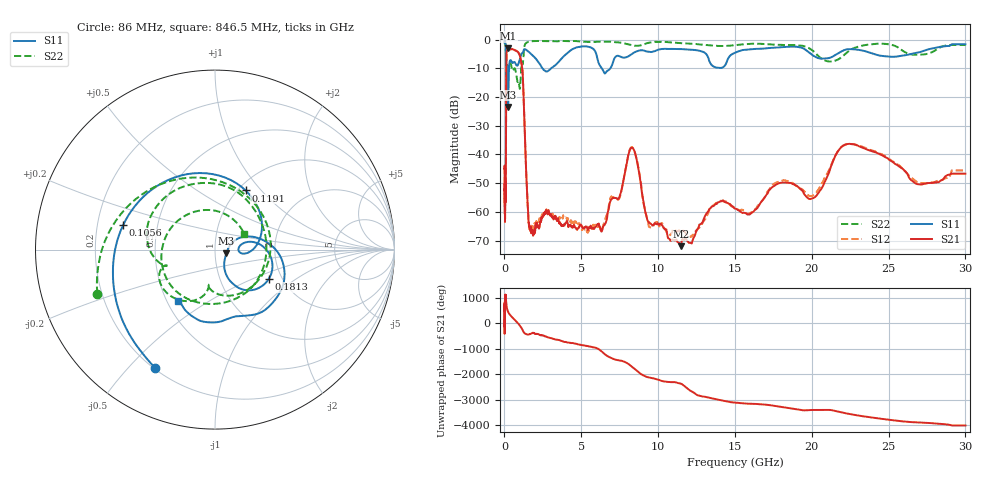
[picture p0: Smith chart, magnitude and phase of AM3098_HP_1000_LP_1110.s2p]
! Date/Time: Thu, Feb 28, 2019 8:40 AM
! Network Analyzer: Agilent Technologies E8364B Rev: A.07.50.67
! Sweep from 0.010 to 30.000 GHz, 1601 Points, Sweep Type: LOG
! Power Supply: 5.023 V, 0.002 A
# Hz S DB R 50
!freq MagS11 AngS11 MagS21 AngS21 MagS12 AngS12 MagS22 AngS22
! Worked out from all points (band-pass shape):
!   1601 points, 10 MHz to 30 GHz, reference 50 ohm
!   highest |S21| = -3.10 dB at 254.7 MHz (marker M1); lowest = -71.9 dB at 11.48 GHz (marker M2)
!   |S21| within 3 dB of the highest: 128 MHz to 1.025 GHz (897.3 MHz wide, 156 % of centre)
!   lowest |S11| = -23.5 dB at 238.7 MHz (marker M3), VSWR 1.14, Z = 56.7 - j2.45 ohm
!   |S11| at or under -10 dB: 192.4 MHz to 298.8 MHz (106.4 MHz wide, 43.3 % of centre); 2.473 GHz to 3.035 GHz (562.5 MHz wide, 20.4 % of centre); 6.333 GHz to 6.896 GHz (563.8 MHz wide, 8.52 % of centre)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
!   |S22| runs from -17.2 to -0.5 dB; largest |S21 - S12| = 0.012
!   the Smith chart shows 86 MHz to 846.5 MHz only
!   S11 on the Smith chart (normalised r, x): 86 MHz: 0.21, -0.60; 105.6 MHz: 0.31, +0.12; 119.1 MHz: 1.08, +0.83; 181.3 MHz: 1.71, -0.63; 846.5 MHz: 0.57, -0.38
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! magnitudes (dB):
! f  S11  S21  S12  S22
! 10 MHz  -0.3  -45.1  -44.5  -0.6
! 38.04 MHz  -0.5  -59.7  -59.3  -1.0
! 86 MHz  -2.6  -51.4  -50.7  -3.1
! 105.6 MHz  -5.5  -26.4  -26.5  -7.2
! 119.1 MHz  -8.6  -10.3  -10.3  -10.5
! 144.7 MHz  -16.9  -4.3  -4.2  -13.2
! 181.3 MHz  -9.3  -3.7  -3.7  -8.8
! 238.7 MHz  -23.5  -3.1  -3.1  -10.9
! 254.7 MHz  -18.7  -3.1  -3.1  -10.5
! 550.5 MHz  -8.1  -3.4  -3.4  -10.8
! 846.5 MHz  -9.1  -4.2  -4.2  -14.7
! 1.178 GHz  -4.7  -11.3  -11.3  -8.7
! 1.614 GHz  -4.4  -64.7  -65.8  -0.8
! 2.084 GHz  -6.9  -65.2  -63.4  -0.5
! 6.202 GHz  -9.0  -65.2  -65.0  -0.7
! 7.926 GHz  -6.2  -44.1  -43.8  -1.5
! 8.416 GHz  -4.6  -38.3  -38.3  -2.1
! 9.396 GHz  -4.3  -63.5  -65.0  -1.1
! 11.48 GHz  -3.3  -71.9  -66.5  -1.3
! 20.1 GHz  -5.6  -55.2  -54.2  -4.1
! 22.56 GHz  -3.3  -36.3  -36.4  -3.5
! 30 GHz  -1.7  -46.7  -45.5  -1.9
